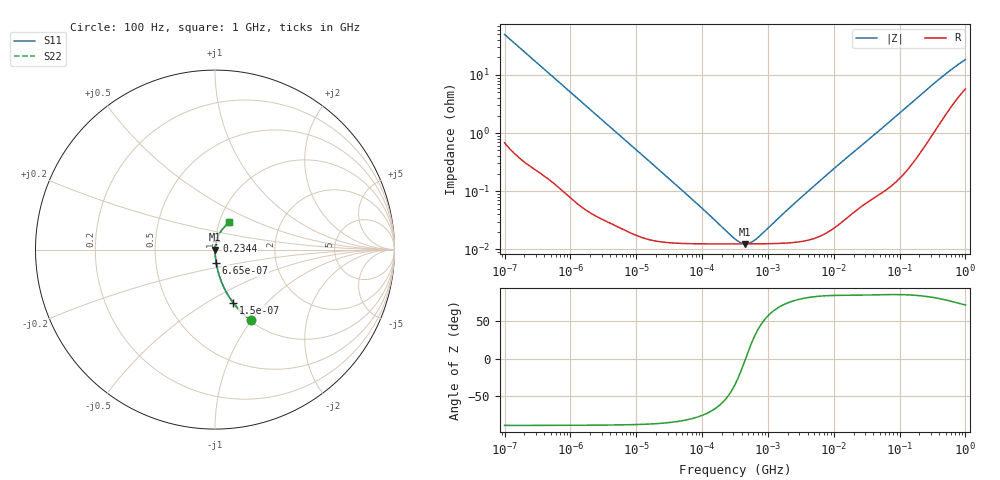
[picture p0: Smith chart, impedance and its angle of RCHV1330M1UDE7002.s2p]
! RCHV1330M1UDE7002  S-PARAMETER MODEL  (AEC-Q200 qualified)
! Model Generated by ELNA Corporation (http://www.ty-top.com)
! Version 1.0
! ELNA Control No. 240229
! Copyright (c) 2024 ELNA CO.,LTD. All Rights Reserved.
! Products Name : CONDUCTIVE POLYMER HYBRID ALUMINUM ELECTROLYTIC CAPACITORS
! Characteristics :
!  Capacitance  :  33uF  ,  Rated voltage  :  50V
!  Operating Temp. Range  :  -55 to +105 degC  ,  Endurance  :  5000hr at 105 degC
!  Dimension D  :  6.3mm  ,  Dimension L  :  7.7mm
! Frequency Range : 100Hz - 1GHz
! External Node Assignments :
!  1  o---| |---o  2
# MHz S RI R 50
!Freq[MHz].  S11 Real  S11 Imag  S21 Real  S21 Imag  S12 Real  S12 Imag  S22 Real  S22 Imag
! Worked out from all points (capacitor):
!   401 points, 100 Hz to 1 GHz, reference 50 ohm
!   read as one part in series: C = 32.1 uF near 108 Hz
!   lowest |Z| = 12.4 mohm at 454.5 kHz (marker M1)
!   series resonance near 458.3 kHz, so ESL is about 3.8 nH
!   S11 on the Smith chart (normalised r, x): 100 Hz: 1.01, -0.99; 150 Hz: 1.01, -0.66; 665 Hz: 1.00, -0.15; 234.4 MHz: 1.01, +0.10; 1 GHz: 1.11, +0.35
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0.0001  0.2005 -0.3936  0.7995 0.3936  0.7995 0.3936  0.2005 -0.3936
0.00015  0.102 -0.2965  0.898 0.2965  0.898 0.2965  0.102 -0.2965
0.000198  0.0616 -0.2342  0.9384 0.2342  0.9384 0.2342  0.0616 -0.2342
0.000309  0.0274 -0.1564  0.9726 0.1564  0.9726 0.1564  0.0274 -0.1564
0.000665  0.0068 -0.0749  0.9932 0.0749  0.9932 0.0749  0.0068 -0.0749
0.001488  0.00168 -0.0339  0.9983 0.0339  0.9983 0.0339  0.00168 -0.0339
0.004241  0.000416 -0.012  0.9996 0.012  0.9996 0.012  0.000416 -0.012
0.022131  0.000141 -0.00232  0.9999 0.00232  0.9999 0.00232  0.000141 -0.00232
0.090678  0.000124 -0.000546  0.9999 0.000546  0.9999 0.000546  0.000124 -0.000546
0.316228  0.000123 -8.54e-05  0.9999 8.54e-05  0.9999 8.54e-05  0.000123 -8.54e-05
0.386812  0.000123 -3.83e-05  0.9999 3.83e-05  0.9999 3.83e-05  0.000123 -3.83e-05
0.454465  0.000124 -1.85e-06  0.9999 1.85e-06  0.9999 1.85e-06  0.000124 -1.85e-06
0.555904  0.000124 4.38e-05  0.9999 -4.38e-05  0.9999 -4.38e-05  0.000124 4.38e-05
0.679986  0.000124 9.12e-05  0.9999 -9.12e-05  0.9999 -9.12e-05  0.000124 9.12e-05
1.938653  0.000128 0.000449  0.9999 -0.000449  0.9999 -0.000449  0.000128 0.000449
4.704354  0.000151 0.00114  0.9998 -0.00114  0.9998 -0.00114  0.000151 0.00114
12.37371  0.000283 0.00296  0.9997 -0.00296  0.9997 -0.00296  0.000283 0.00296
69.9842  0.00139 0.0154  0.9986 -0.0154  0.9986 -0.0154  0.00139 0.0154
234.4229  0.00808 0.0497  0.9919 -0.0497  0.9919 -0.0497  0.00808 0.0497
546.3866  0.0343 0.1033  0.9657 -0.1033  0.9657 -0.1033  0.0343 0.1033
817.523  0.0617 0.1356  0.9383 -0.1356  0.9383 -0.1356  0.0617 0.1356
1000  0.0791 0.1517  0.9209 -0.1517  0.9209 -0.1517  0.0791 0.1517
